[IBIS VER]   5.0
[File Name]   am13e230pzg.ibs
[File Rev]   1.0
[Date]   February 08, 2026
[Source]   File originated at Texas Instruments
[Copyright]   (c) 2012, Texas Instruments Inc.
[Component]   am13e230pzg
[Manufacturer] Texas Instruments
[Package]
| Variable   Typ   Min   Max
   R_pkg 3.31E-01 1.79E-01 4.09E-01
   L_pkg 6.96E-09 4.29E-09 8.69E-09
   C_pkg 1.96E-14 1.45E-14 4.60E-14
[Pin]   signal_name   model_name   R_pin   L_pin   C_pin
   1   PC2   BCF3385DSHYPBFZSD_87U 3.83E-01 8.46E-09 3.97E-14
   2   PC3   BCF3385DSHYPBFZSD_87U 3.62E-01 8.13E-09 1.93E-14
   3   PC4   BCF3385DSHYPBFZSD_87U 3.50E-01 7.91E-09 1.88E-14
   4   PC5   BCF3385DSHYPBFZSD_87U 3.41E-01 7.70E-09 1.83E-14
   5   PC6   BCF3385DSWHYPBFZSD_87U 3.34E-01 7.52E-09 1.78E-14
   6   VDD   NC 3.34E-01 7.42E-09 1.74E-14
   7   PB13   BCF3385DSWHYPBFZSD_87U 3.26E-01 7.22E-09 1.70E-14
   8   PB14   BCF3385DSHYPBFZSD_87U 3.24E-01 7.10E-09 1.66E-14
   9   PB15   BCF3385DSHYPBFZSD_87U 3.23E-01 6.98E-09 1.61E-14
   10   PC25   BCF3385DSHYPBFZSD_87U 3.25E-01 6.89E-09 1.58E-14
   11   PC26   BCF3385DSHYPBFZSD_87U 3.24E-01 6.77E-09 1.53E-14
   12 PC16_X1   BCF3385DSHYPBFZSD_87U 3.24E-01 6.67E-09 1.81E-14
   13 PC17_X2   BCF3385DSHYPBFZSD_87U 3.22E-01 6.54E-09 1.76E-14
   14   NRST   BQ0491FSSD_XRSN_87U 3.25E-01 6.67E-09 1.81E-14
   15   PB0   BCF3385DSHYPBFZSD_87U 3.27E-01 6.80E-09 1.54E-14
   16   PB1   BCF3385DSWHYPBFZSD_87U 3.30E-01 6.94E-09 1.58E-14
   17   PB2   BCF3385DSHYPBFZSD_87U 3.34E-01 7.09E-09 1.62E-14
   18   PB3   BCF3385DSHYPBFZSD_87U 3.40E-01 7.26E-09 1.67E-14
   19   PC18   BCF3385DSHYPBFZSD_87U 3.31E-01 7.28E-09 1.70E-14
   20   PA0   BCF3385DSWHYPBFZSD_87U 3.37E-01 7.45E-09 1.75E-14
   21   PA1   BCF3385DSHYPBFZSD_87U 3.44E-01 7.63E-09 1.79E-14
   22   PA2   BCF3385DSWHYPBFZSD_87U 3.53E-01 7.83E-09 1.84E-14
   23   VSSA   NC 2.00E-01 6.35E-09 2.15E-14
   24   VDDA   NC 2.04E-01 6.51E-09 2.21E-14
   25   PA3   BCF3385DSHYPBFZSD_87U 3.83E-01 8.46E-09 3.97E-14
   26   PA4   BCF3385DSHYPBFZSD_87U 3.90E-01 8.52E-09 3.97E-14
   27   PA5   BCF3385DSHYPBFZSD_87U 3.75E-01 8.25E-09 1.93E-14
   28   PA6   BCF3385DSHYPBFZSD_87U 3.61E-01 8.01E-09 1.88E-14
   29   PA7   BCF3385DSHYPBFZSD_87U 3.49E-01 7.78E-09 1.83E-14
   30   PB4   BCF3385DSHYPBFZSD_87U 3.39E-01 7.57E-09 1.78E-14
   31   PB5   BCF3385DSWHYPBFZSD_87U 3.31E-01 7.38E-09 1.74E-14
   32   PA16   BCF3385DSHYPBFZSD_87U 3.25E-01 7.21E-09 1.69E-14
   33   PA17   BCF3385DSHYPBFZSD_87U 3.20E-01 7.05E-09 1.65E-14
   34   PA18   BCF3385DSHYPBFZSD_87U 3.16E-01 6.90E-09 1.61E-14
   35   VREFLO   NC 3.16E-01 6.79E-09 1.57E-14
   36   VREFHI   NC 3.16E-01 6.68E-09 1.53E-14
   37   VDDA   NC 3.20E-01 6.62E-09 1.80E-14
   38   PC7   BCF3385DSHYPBFZSD_87U 3.20E-01 6.51E-09 1.75E-14
   39   PC8   BCF3385DSHYPBFZSD_87U 3.15E-01 6.35E-09 1.70E-14
   40   PC9   BCF3385DSHYPBFZSD_87U 3.11E-01 6.21E-09 1.65E-14
   41   PC10   BCF3385DSHYPBFZSD_87U 3.09E-01 6.08E-09 1.59E-14
   42   PC11   BCF3385DSHYPBFZSD_87U 3.08E-01 5.96E-09 1.54E-14
   43   PC12   BCF3385DSHYPBFZSD_87U 3.09E-01 5.86E-09 1.49E-14
   44   PC13   BCF3385DSHYPBFZSD_87U 3.11E-01 6.15E-09 1.45E-14
   45   PC14   BCF3385DSHYPBFZSD_87U 3.16E-01 6.07E-09 2.16E-14
   46   PC15   BCF3385DSHYPBFZSD_87U 3.22E-01 6.01E-09 2.08E-14
   47   PA26   BCF3385DSHYPBFZSD_87U 3.29E-01 5.97E-09 2.00E-14
   48   VSS   NC 1.79E-01 4.29E-09 2.18E-14
   49   VDD   NC 3.48E-01 5.91E-09 1.85E-14
   50   PA27   BCF3385DSHYPBFZSD_87U 3.63E-01 6.08E-09 3.56E-14
   51   PA28   BCF3385DSHYPBFZSD_87U 3.84E-01 8.47E-09 3.97E-14
   52   PA29   BCF3385DSHYPBFZSD_87U 3.71E-01 8.22E-09 1.93E-14
   53   PA30   BCF3385DSHYPBFZSD_87U 3.59E-01 8.00E-09 1.88E-14
   54   PA31   BCF3385DSHYPBFZSD_87U 3.49E-01 7.79E-09 1.84E-14
   55   PB24   BCF3385DSHYPBFZSD_87U 3.44E-01 7.62E-09 1.79E-14
   56   PB25   BCF3385DSHYPBFZSD_87U 3.37E-01 7.45E-09 1.75E-14
   57   PB26   BCF3385DSHYPBFZSD_87U 3.32E-01 7.29E-09 1.70E-14
   58   PB27   BCF3385DSHYPBFZSD_87U 3.28E-01 7.14E-09 1.66E-14
   59   PB28   BCF3385DSHYPBFZSD_87U 3.26E-01 7.01E-09 1.62E-14
   60   PB29   BCF3385DSHYPBFZSD_87U 3.24E-01 6.89E-09 1.58E-14
   61   PB30   BCF3385DSHYPBFZSD_87U 3.23E-01 6.77E-09 1.53E-14
   62   PB31   BCF3385DSHYPBFZSD_87U 3.24E-01 6.67E-09 1.81E-14
   63   VSS   NC 3.31E-01 6.64E-09 1.77E-14
   64   VDD   NC 3.35E-01 6.78E-09 1.82E-14
   65   PB6   BCF3385DSHYPBFZSD_87U 3.34E-01 6.88E-09 1.54E-14
   66   PB7   BCF3385DSHYPBFZSD_87U 3.40E-01 7.04E-09 1.59E-14
   67   PB8   BCF3385DSHYPBFZSD_87U 3.36E-01 7.11E-09 1.62E-14
   68   PB9   BCF3385DSHYPBFZSD_87U 3.42E-01 7.28E-09 1.67E-14
   69   PA8   BCF3385DSHYPBFZSD_87U 3.50E-01 7.47E-09 1.72E-14
   70   PA9   BCF3385DSHYPBFZSD_87U 3.59E-01 7.67E-09 1.76E-14
   71   PA10   BCF3385DSHYPBFZSD_87U 3.70E-01 7.89E-09 1.81E-14
   72   PA11   BCF3385DSHYPBFZSD_87U 3.65E-01 7.95E-09 1.85E-14
   73   PA12  BCPF335585DSHYPBFZSD_87U 3.77E-01 8.18E-09 1.90E-14
   74   VSS   NC 3.95E-01 8.48E-09 1.95E-14
   75   VDD   NC 2.22E-01 6.80E-09 4.60E-14
   76   PA13 BCF3385DSHYPBFZSD_TMS_87U 4.06E-01 8.69E-09 3.99E-14
   77   PA14 BCF3385DSHYPBFZSD_TMS_87U 3.59E-01 8.09E-09 1.92E-14
   78   PA15  BCPF335585DSHYPBFZSD_87U 3.47E-01 7.86E-09 1.87E-14
   79   PB10   BCF3385DSHYPBFZSD_87U 3.37E-01 7.65E-09 1.82E-14
   80   PB11   BCF3385DSHYPBFZSD_87U 3.29E-01 7.46E-09 1.78E-14
   81   PB12   BCF3385DSHYPBFZSD_87U 3.22E-01 7.29E-09 1.73E-14
   82   PB16   BCF3385DSHYPBFZSD_87U 3.26E-01 7.21E-09 1.69E-14
   83   PB17   BCF3385DSHYPBFZSD_87U 3.20E-01 7.05E-09 1.65E-14
   84   PB18  BCPF335585DSHYPBFZSD_87U 3.20E-01 6.94E-09 1.61E-14
   85   PB19   BCF3385DSWHYPBFZSD_87U 3.18E-01 6.81E-09 1.57E-14
   86   PB20   BCF3385DSHYPBFZSD_87U 3.15E-01 6.68E-09 1.53E-14
   87   PB21   BCF3385DSHYPBFZSD_87U 3.14E-01 6.56E-09 1.80E-14
   88   PB22   BCF3385DSHYPBFZSD_87U 3.14E-01 6.45E-09 1.75E-14
   89   PB23   BCF3385DSHYPBFZSD_87U 3.14E-01 6.34E-09 1.70E-14
   90   PA19  BCPF335585DSHYPBFZSD_87U 3.15E-01 6.25E-09 1.65E-14
   91   PA20   BCF3385DSHYPBFZSD_87U 3.18E-01 6.17E-09 1.60E-14
   92   PA21   BCF3385DSHYPBFZSD_87U 3.18E-01 6.06E-09 1.55E-14
   93   PA22   BCF3385DSHYPBFZSD_87U 3.22E-01 6.00E-09 1.50E-14
   94   PA23   BCF3385DSHYPBFZSD_87U 3.28E-01 6.32E-09 1.46E-14
   95   PA24   BCF3385DSHYPBFZSD_87U 3.33E-01 6.24E-09 2.17E-14
   96   PA25   BCF3385DSHYPBFZSD_87U 3.41E-01 6.21E-09 2.10E-14
   97   PC0   BCF3385DSHYPBFZSD_87U 3.51E-01 6.19E-09 2.02E-14
   98   PC1   BCF3385DSHYPBFZSD_87U 3.64E-01 6.19E-09 1.95E-14
   99   VSS   NC 1.97E-01 4.35E-09 2.15E-14
   100   VDD   NC 3.96E-01 6.42E-09 3.61E-14
| End of package information
|   Component BCF3385DSHYPBFZSD_87U
[Component] BCF3385DSHYPBFZSD_87U
[Manufacturer] Texas Instruments
[Package]
| variable   typ   min   max
R_pkg   0.0   0.0   0.0
L_pkg   0.0H   0.0H   0.0H
C_pkg   0.0F   0.0F   0.0F
[Pin]  signal_name   model_name   R_pin   L_pin   C_pin
PAD   PAD   BCF3385DSHYPBFZSD_87U
VDDS   VDDS   Power
VSS   VSS   Gnd
A   A   NC
GZ   GZ   NC
[Model Selector] BCF3385DSHYPBFZSD_87U
BCF3385DSHYPBFZSD_87U_PUPDOFF PI=1 PSEL=1
BCF3385DSHYPBFZSD_87U_PDON PI=0 PSEL=0
BCF3385DSHYPBFZSD_87U_PUON PI=0 PSEL=1
|   Component BCF3385DSHYPBFZSD_TMS_87U
[Component] BCF3385DSHYPBFZSD_TMS_87U
[Manufacturer] Texas Instruments
[Package]
| variable   typ   min   max
R_pkg   0.0   0.0   0.0
L_pkg   0.0H   0.0H   0.0H
C_pkg   0.0F   0.0F   0.0F
[Pin]  signal_name   model_name   R_pin   L_pin   C_pin
PAD   PAD   BCF3385DSHYPBFZSD_TMS_87U
VDDS   VDDS   Power
VSS   VSS   Gnd
A   A   NC
GZ   GZ   NC
[Model Selector] BCF3385DSHYPBFZSD_TMS_87U
BCF3385DSHYPBFZSD_TMS_87U_PUPDOFF PI=1 PSEL=1
BCF3385DSHYPBFZSD_TMS_87U_PDON PI=0 PSEL=0
BCF3385DSHYPBFZSD_TMS_87U_PUON PI=0 PSEL=1
|   Component BCF3385DSWHYPBFZSD_87U
[Component] BCF3385DSWHYPBFZSD_87U
[Manufacturer] Texas Instruments
[Package]
| variable   typ   min   max
R_pkg   0.0   0.0   0.0
L_pkg   0.0H   0.0H   0.0H
C_pkg   0.0F   0.0F   0.0F
[Pin]  signal_name   model_name   R_pin   L_pin   C_pin
PAD   PAD   BCF3385DSWHYPBFZSD_87U
VDDS   VDDS   Power
VSS   VSS   Gnd
A   A   NC
GZ   GZ   NC
[Model Selector] BCF3385DSWHYPBFZSD_87U
BCF3385DSWHYPBFZSD_87U_PUPDOFF PI=1 PSEL=1
BCF3385DSWHYPBFZSD_87U_PDON PI=0 PSEL=0
BCF3385DSWHYPBFZSD_87U_PUON PI=0 PSEL=1
|   Component BCPF335585DSHYPBFZSD_87U
[Component] BCPF335585DSHYPBFZSD_87U
[Manufacturer] Texas Instruments
[Package]
| variable   typ   min   max
R_pkg   0.0   0.0   0.0
L_pkg   0.0H   0.0H   0.0H
C_pkg   0.0F   0.0F   0.0F
[Pin]  signal_name   model_name   R_pin   L_pin   C_pin
PAD   PAD   BCPF335585DSHYPBFZSD_87U
VDDS   VDDS   Power
VSS   VSS   Gnd
A   A   NC
GZ   GZ   NC
[Model Selector] BCPF335585DSHYPBFZSD_87U
BCPF335585DSHYPBFZSD_87U_PUPDOFF_D0 DS=0
BCPF335585DSHYPBFZSD_87U_PUPDOFF_D1 DS=1
BCPF335585DSHYPBFZSD_87U_PDON PI=0 PSEL=0
BCPF335585DSHYPBFZSD_87U_PUON PI=0 PSEL=1
|   Component BQ0491FSSD_XRSN_87U
[Component] BQ0491FSSD_XRSN_87U
[Manufacturer] Texas Instruments
[Package]
| variable   typ   min   max
R_pkg   0.0   0.0   0.0
L_pkg   0.0H   0.0H   0.0H
C_pkg   0.0F   0.0F   0.0F
[Pin]  signal_name   model_name   R_pin   L_pin   C_pin
PAD   PAD   BQ0491FSSD_XRSN_87U
VDDS   VDDS   Power
VSS   VSS   Gnd
A   A   NC
[Model Selector] BQ0491FSSD_XRSN_87U
BQ0491FSSD_XRSN_87U_PUPDOFF PI=1
BQ0491FSSD_XRSN_87U_PUPDON PI=0
| Models and submodels in the file (15): BCF3385DSHYPBFZSD_87U_PUPDOFF (I/O), BCF3385DSHYPBFZSD_87U_PDON (Input), BCF3385DSHYPBFZSD_87U_PUON (Input), BCF3385DSHYPBFZSD_TMS_87U_PUPDOFF (I/O), BCF3385DSHYPBFZSD_TMS_87U_PDON (Input), BCF3385DSHYPBFZSD_TMS_87U_PUON (Input), BCF3385DSWHYPBFZSD_87U_PUPDOFF (I/O), BCF3385DSWHYPBFZSD_87U_PDON (Input), BCF3385DSWHYPBFZSD_87U_PUON (Input), BCPF335585DSHYPBFZSD_87U_PUPDOFF_D0 (I/O), BCPF335585DSHYPBFZSD_87U_PUPDOFF_D1 (I/O), BCPF335585DSHYPBFZSD_87U_PDON (Input), BCPF335585DSHYPBFZSD_87U_PUON (Input), BQ0491FSSD_XRSN_87U_PUPDOFF (Input), BQ0491FSSD_XRSN_87U_PUPDON (Input)
